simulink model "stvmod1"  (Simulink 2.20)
settings: Solver=FixedStepDiscrete  StartTime=0.0  StopTime=800  MaxStep=0.01  RelTol=1e-3  AbsTol=1e-6

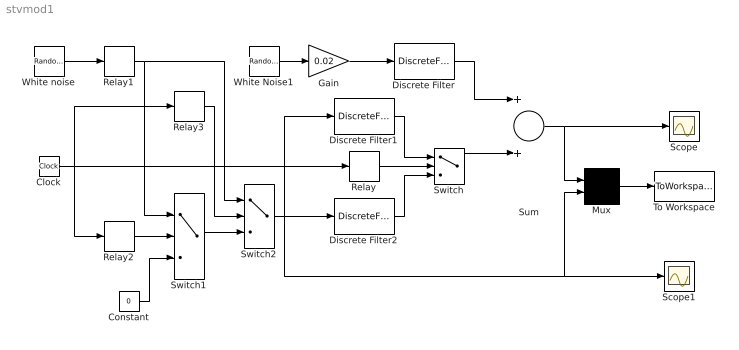
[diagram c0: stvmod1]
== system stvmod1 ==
  Clock : Clock
  Constant : Constant  Value=0
  Discrete Filter : DiscreteFilter  Numerator=[1]  Denominator=[1 -0.9]  SampleTime=-1
  Discrete Filter1 : DiscreteFilter  Numerator=[0.1]  Denominator=[1 -0.9]  SampleTime=1
  Discrete Filter2 : DiscreteFilter  Numerator=[0.5]  Denominator=[1 -0.9]  SampleTime=1
  Gain : Gain  Gain=0.02
  Mux : Mux  Inputs=2
  Relay : Relay  OnSwitchValue=500  OffSwitchValue=500  OnOutputValue=-1  OffOutputValue=1
  Relay1 : Relay  OnSwitchValue=0  OffSwitchValue=0  OnOutputValue=1  OffOutputValue=-1
  Relay2 : Relay  OnSwitchValue=200  OffSwitchValue=200  OnOutputValue=-1  OffOutputValue=1
  Relay3 : Relay  OnSwitchValue=400  OffSwitchValue=400  OnOutputValue=1  OffOutputValue=-1
  Scope : Scope
  Scope1 : Scope
  Sum : Sum  Inputs=++
  Switch : Switch  Threshold=0
  Switch1 : Switch  Threshold=0
  Switch2 : Switch  Threshold=0
  To Workspace : ToWorkspace  VariableName=ut  SampleTime=-1
  White noise : RandomNumber  Mean=0  Variance=0.02  Seed=9  SampleTime=0
  White Noise1 : RandomNumber  Mean=0  Variance=0.02  Seed=201  SampleTime=0
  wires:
  Relay2/1 -> Switch1/2
  Constant/1 -> Switch1/3
  Switch1/1 -> Switch2/3
  Relay3/1 -> Switch2/2
  White noise/1 -> Relay1/1
  Relay1/1 -> Switch2/1, Switch1/1
  Clock/1 -> Relay/1, Relay3/1, Relay2/1
  Switch2/1 -> Scope1/1, Mux/2, Discrete Filter2/1, Discrete Filter1/1
  Sum/1 -> Scope/1, Mux/1
  Mux/1 -> To Workspace/1
  Relay/1 -> Switch/2
  Switch/1 -> Sum/2
  Discrete Filter/1 -> Sum/1
  Gain/1 -> Discrete Filter/1
  White Noise1/1 -> Gain/1
  Discrete Filter2/1 -> Switch/3
  Discrete Filter1/1 -> Switch/1
